PROGRAM MAIN
VAR
	eComState 				: E_ComState;
	
	(* slave *)
	AODB					: ARRAY[0..10] OF ST_IEC870_5_101AODBEntry; // Application object data base
	hServer					: T_HSERVER;
	fbSlave					: FB_IEC870_5_104Slave;
	
	fbValueManipTime		: TON;			// time for value manipulation - example
END_VAR

CASE eComState OF
INIT:
// INIT slave
	// TCP/IP server handle
	F_CreateServerHnd( 	'', 					// own TwinCAT netID, empty string = local
						'127.0.0.1',			// own (slave) IP address
						2404,					// communication port - check firewall settings
						LISTEN_MODE_CLOSEALL OR CONNECT_MODE_ENABLEDBG, // close all previous opened socket connections and enable debug output
						TRUE,					// enable connection
						hServer );			

	// system parameter					
	fbSlave.sysPara.asduAddr 		:= 3;		// common ASDU address
	fbSlave.sysPara.dbgMode 		:= IEC870_DEBUGMODE_DEVSTATE  OR IEC870_DEBUGMODE_LINKERROR;(*OR IEC870_DEBUGMODE_ASDU OR IEC870_DEBUGMODE_LINKLAYER*)(* enable output of device state change messages *)
	fbSlave.sysPara.bSyncTime		:= TRUE;	// sync IEC system time after reception of C_CS_NA_1 commmando
	fbSlave.sysPara.bSyncPCTime 	:= TRUE; 	// sync PC time from master
	fbSlave.sysPara.tSyncToPCTime	:= T#30S;
	
// INIT data points
	// SLAVE -> MASTER (monitoring direction)

		(* bSlaveToMaster *)
		F_iecInitAOEntry( 	M_SP_NA_1,			// type is single point
							10,					// information object address
							IEC870_GRP_INROGEN, // general interrogation group and spontaneous data transmission
							0,					// multiplier - not used
							MAP_AREA_MEMORY,	// map this datapoint FROM PLC memory area (buffer)
							0,					// map FROM byte offset		AT%MX0.0 -> 0 byte offset
							0,					// map FROM bit offset		AT%MX0.0 -> 0 bit offset
							AODB[0] );			//data base array element
							
		(* nBitstring *)					
		F_iecInitAOEntry(	M_BO_TB_1,			// type is bitstring (32Bit)
							11,					// information object address
							IEC870_GRP_INROGEN, // general interrogation group and spontaneous data transmission
							0,					// multiplier - not used 
							MAP_AREA_MEMORY,	// map this datapoint FROM PLC memory area (buffer)
							4,					// map FROM byte offset		AT%MD1 -> 4*1 byte offset
							0,					// map FROM bit offset
							AODB[1] );			//data base array element

		(* nMeasurementValue *)					
		F_iecInitAOEntry(	M_ME_NB_1,			// type is measured value, scaled
							12,					// information object address
							IEC870_GRP_INROGEN, // general interrogation group and spontaneous data transmission
							0,					// multiplier - not used 
							MAP_AREA_MEMORY,	// map this datapoint FROM PLC memory area (buffer)
							20,					// map FROM byte offset		AT%MW10 -> 2*10 byte offset
							0,					// map FROM bit offset
							AODB[2] );			//data base array element

		(* fMeasurementValue *)					
		F_iecInitAOEntry(	M_ME_NC_1,			// type is measured value, short floating point
							13,					// information object address
							IEC870_GRP_INROGEN, // general interrogation group and spontaneous data transmission
							0,					// multiplier - not used 
							MAP_AREA_MEMORY,	// map this datapoint FROM PLC memory area (buffer)
							24,					// map FROM byte offset		AT%MD6 -> 4*6 byte offset
							0,					// map FROM bit offset
							AODB[3] );			//data base array element

		(* nCounter*)
		F_iecInitAOEntry(	M_IT_NA_1,			// type is integrated total
							200,				// information object address
							IEC870_GRP_REQCOGEN OR IEC870_GRP_LOCFREEZE,	// general counter interrogation
							0,					// multiplier - not used 
							MAP_AREA_MEMORY,	// map this datapoint FROM PLC memory area (buffer)
							40,					// map FROM byte offset		AT%MD10 -> 4*10 byte offset
							0,					// map FROM bit offset
							AODB[4] );			//data base array element
							
							
	//MASTER -> SLAVE (control directon)	

		(* bMasterToSlave - single point in command direction *)
		F_iecInitAOEntry(	C_SC_NA_1,			// type is single command
							101, 				// information object address
							0,  				// group - not used
							0, 					// multiplier - not used 
							MAP_AREA_MEMORY, 	// map this datapoint TO PLC memory area (buffer)
							100, 				// map TO byte offset		AT%MX100.0 -> 100 byte offset
							0, 					// map TO bit offset		AT%MX100.0 -> 0 bit offset
							AODB[10] );			// data base array element				

	eComState := COMMUNICATION;
		
COMMUNICATION:	// INIT completed

	(* execute IEC slave function block *)
	fbSlave( bEnable 	:= TRUE,
			hServer 	:= hServer, 		// server connection handle
			pAOEntries 	:= ADR(AODB),
			cbAOEntries := SIZEOF(AODB),		
			pInputs 	:= 0,				// intput buffer where the data point values are mapped to and from
			cbInputs	:= 0,				(* not used in this example project *)
			pOutputs 	:= 0,				// output buffer where the data point values are mapped to and from
			cbOutputs 	:= 0,				(* not used in this example project *)	
			pMemory 	:= ADR(memory),		// memory buffer where the data point values are mapped to and from
			cbMemory 	:= SIZEOF(memory),
			pData 		:= 0,				// data buffer where the data point values are mapped to and from
			cbData 		:= 0 );				(* not used in this example project *)


	(* Check for device errors, remove them and log message to the TwinCAT System Manager log view *)
	REPEAT
		fbSlave.system.device.errors.RemoveError();
		IF fbSlave.system.device.errors.bOk THEN
			ADSLOGSTR( ADSLOG_MSGTYPE_ERROR OR ADSLOG_MSGTYPE_LOG, 'IEC60870-5-104 slave error: 0x%s',
						DWORD_TO_HEXSTR( fbSlave.system.device.errors.getError.nErrId, 8, FALSE) );
		END_IF
	UNTIL NOT fbSlave.system.device.errors.bOk
	END_REPEAT

END_CASE


// value manipulation
fbValueManipTime(IN:= NOT fbValueManipTime.Q, PT:= T#1S);
IF fbValueManipTime.Q THEN
	bSlaveToMaster := NOT bSlaveToMaster;
	nBitstring:=nBitstring+1;
	nMeasurementValue:=nMeasurementValue+2;
	fMeasurementValue:=fMeasurementValue+1.5;
	nCounter := nCounter + 10;
END_IF

END_PROGRAM
